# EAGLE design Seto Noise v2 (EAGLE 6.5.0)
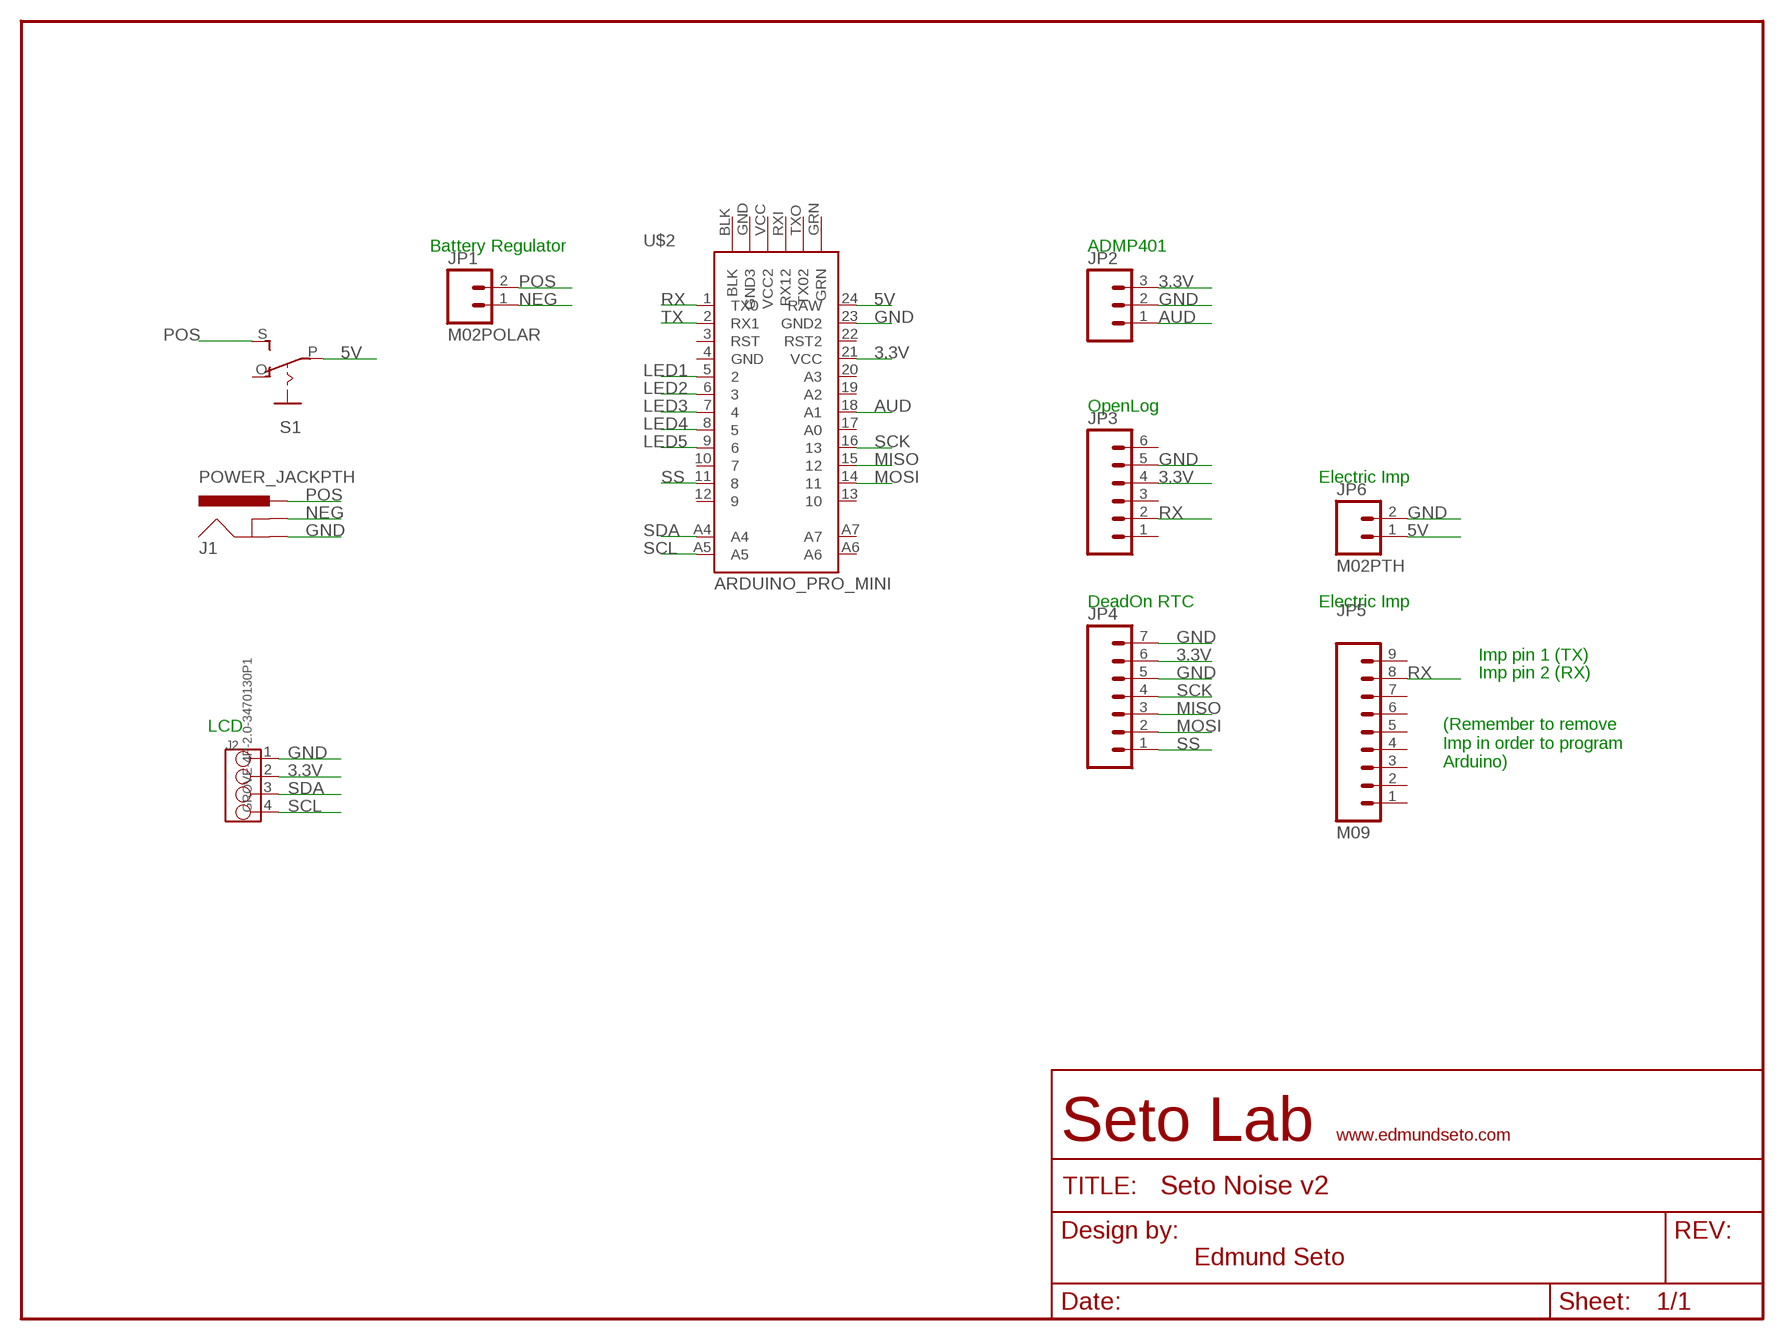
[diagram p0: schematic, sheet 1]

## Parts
J1  POWER_JACKPTH  [POWER_JACK_PTH]
J2  GROVE-4P-2.0-3470130P1  [4P-2.0]
JP1  M02POLAR  [MOLEX-1X2]
JP2  M03PTH  [1X03]
JP3  M06SIP  [1X06]
JP4  M07  [1X07]
JP5  M09  [1X09]
JP6  M02PTH  [1X02]
S1  EG1218S  [EG1218]
U$2  ARDUINO_PRO_MINI  [ARDUINO_PRO_MINI]

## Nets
3.3V: J2.2 JP2.3 JP3.4 JP4.6 U$2.21(VCC)
5V: JP6.1 S1.P U$2.24(RAW)
AUD: JP2.1 U$2.18(A1)
GND: J1.GND J2.1 JP2.2 JP3.5 JP4.5 JP4.7 JP6.2 U$2.23(GND2)
LED1: U$2.5
LED2: U$2.6
LED3: U$2.7
LED4: U$2.8
LED5: U$2.9
MISO: JP4.3 U$2.15
MOSI: JP4.2 U$2.14
NEG: J1.GNDBREAK JP1.1
POS: J1.PWR JP1.2 S1.S
RX: JP3.2 JP5.8 U$2.1(TX0)
SCK: JP4.4 U$2.16
SCL: J2.4 U$2.A5
SDA: J2.3 U$2.A4
SS: JP4.1 U$2.11
TX: U$2.2(RX1)
Unconnected: JP3.1 JP3.3 JP3.6 JP5.1 JP5.2 JP5.3 JP5.4 JP5.5 JP5.6 JP5.7 JP5.9 S1.O U$2.3(RST) U$2.4(GND) U$2.10 U$2.12 U$2.13 U$2.17(A0) U$2.19(A2) U$2.20(A3) U$2.22(RST2) U$2.A6 U$2.A7 U$2.BLK U$2.GND(GND3) U$2.GRN U$2.RXI(RX12) U$2.TXO(TX02) U$2.VCC(VCC2)

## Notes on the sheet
- Battery Regulator | ADMP401
- OpenLog
- Electric Imp
- DeadOn RTC | Electric Imp
- Imp pin 1 (TX)
- Imp pin 2 (RX)
- LCD
- (Remember to remove 
  Imp in order to program 
  Arduino)

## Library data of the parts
J1 = SparkFun-Connectors:POWER_JACK: Power Jack This is the standard 5.5mm barrel jack for power. The PTH is the most common, proven, reliable, footprint. The Slot footprint only works if the mill layer is transmitted to the PCB fab house so be warned. Spark Fun Electronics SKU : PRT-00119 SMT: CONN-08106 Mating wall wart : TOL-00298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
J2 = OPL Eagle Library:GROVE-4P-2.0
JP1 JP6 = SparkFun-Connectors:M02: Standard 2-pin 0.1" header. Use with
JP2 = SparkFun-Connectors:M03: Header 3 Standard 3-pin 0.1" header. Use with straight break away headers (SKU : PRT-00116), right angle break away headers (PRT-00553), swiss pins (PRT-00743), machine pins (PRT-00117), and female headers (PRT-00115). Molex polarized connector foot print use with SKU : PRT-08232 with associated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
JP3 = SparkFun-Connectors:M06: Header 6 Standard 6-pin 0.1" header. Use with straight break away headers (SKU : PRT-00116), right angle break away headers (PRT-00553), swiss pins (PRT-00743), machine pins (PRT-00117), and female headers (PRT-00115). Molex polarized connector foot print use with SKU : PRT-08094 with associated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
JP4 = SparkFun-Connectors:M07: Header 7 Standard 7-pin 0.1" header. Use with straight break away headers (SKU : PRT-00116), right angle break away headers (PRT-00553), swiss pins (PRT-00743), machine pins (PRT-00117), and female headers (PRT-00115). NOTES ON THE VARIANTS LOCK and LOCK_LONGPADS... This footprint was designed to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
JP5 = SparkFun-Connectors:M09: Header 9 Standard 9-pin 0.1" header. Use with straight break away headers (SKU : PRT-00116), right angle break away headers (PRT-00553), swiss pins (PRT-00743), machine pins (PRT-00117), and female headers (PRT-00115).
S1 = adafruit:EG1218: SLIDING SWITCH 0.1" spacing through hole, vertical SPDT slide switch http://www.ladyada.net/library/pcb/eaglelibrary.html
U$2 = SparkFun-Boards_ES:ARDUINO_PRO_MINI

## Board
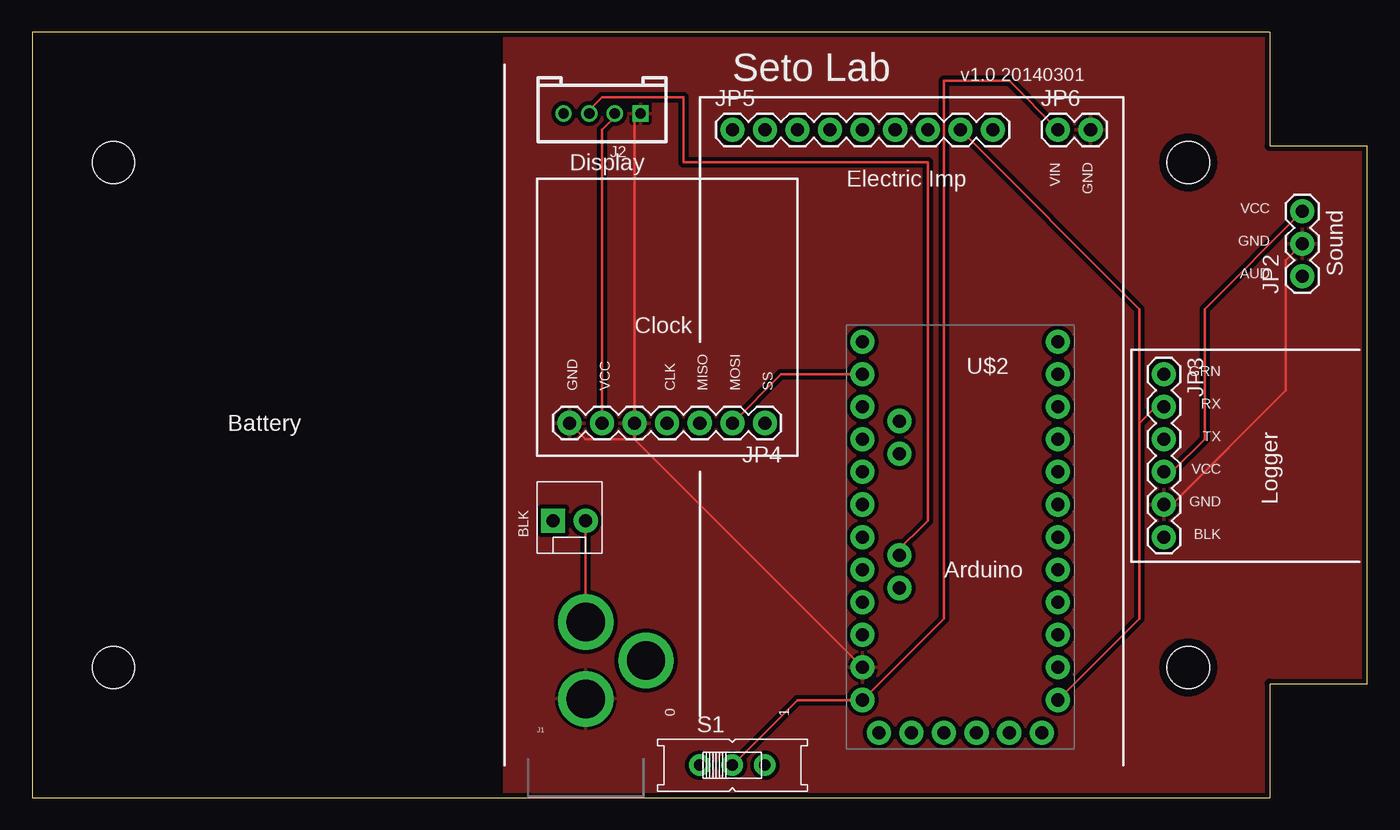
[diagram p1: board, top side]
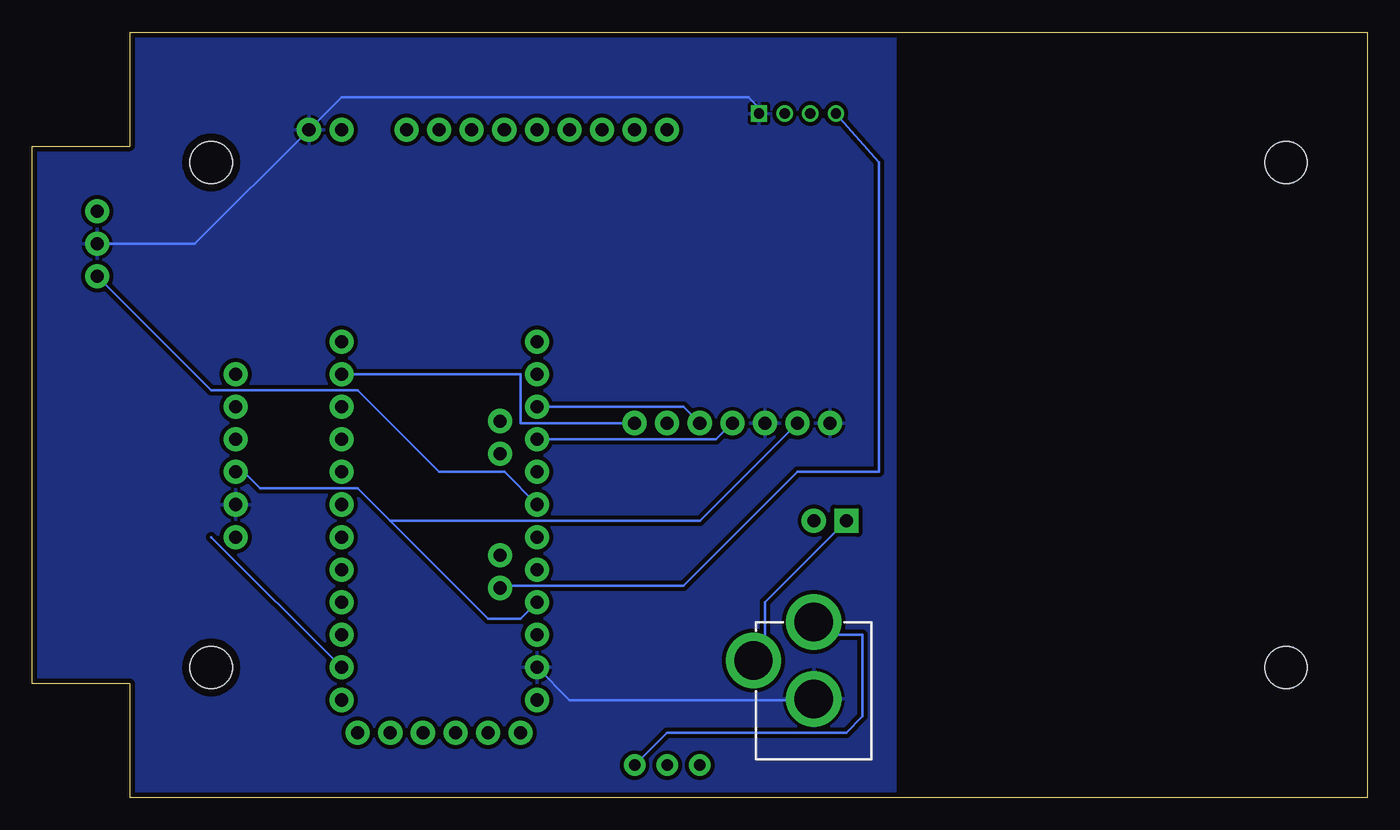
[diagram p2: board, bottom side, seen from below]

Size 104.14 x 59.69 mm. Coordinates in mm from the lower left corner, seen from the top.
Outline: 0,0 96.52,0 96.52,8.89 104.14,8.89 104.14,50.8 96.52,50.8 96.52,59.69 0,59.69 0,0
Copper layers (1*16): Top 0.0356mm / dielectric 1.5011mm / Bottom 0.0356mm
Design rules "LaenPCBOrder": minimum track width 6mil, minimum drill 13mil, track to track 6mil, track to pad 6mil, pad to pad 6mil, via to via 6mil, smd to smd 6mil, copper to edge 15mil, drill to drill 6mil, minimum pad ring 7mil, minimum via ring 7mil, stop-mask expansion 3mil, vias tented up to drill 0mil, thermal gap 10mil

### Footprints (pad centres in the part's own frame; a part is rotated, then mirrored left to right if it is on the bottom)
POWER_JACK_PTH = drill 2.997 pad 4.318: GND 0,7.7; GNDBREAK 4.7,10.7; PWR 0,13.7
4P-2.0 = drill 0.8 pad 1.27 square: 1 -3,0 | drill 0.8 pad 1.27: 2 -1,0; 3 1,0; 4 3,0
MOLEX-1X2 = drill 1.016 pad 1.88 square: 1 0,0 | drill 1.016 pad 1.88: 2 2.54,0
1X03 = drill 1.016 pad 1.88: 1 0,0; 2 2.54,0; 3 5.08,0
1X06 = drill 1.016 pad 1.88: 1 0,0; 2 2.54,0; 3 5.08,0; 4 7.62,0; 5 10.16,0; 6 12.7,0
1X07 = drill 1.016 pad 1.88: 1 0,0; 2 2.54,0; 3 5.08,0; 4 7.62,0; 5 10.16,0; 6 12.7,0; 7 15.24,0
1X09 = drill 1.016 pad 1.88: 1 0,0; 2 2.54,0; 3 5.08,0; 4 7.62,0; 5 10.16,0; 6 12.7,0; 7 15.24,0; 8 17.78,0; 9 20.32,0
1X02 = drill 1.016 pad 1.88: 1 0,0; 2 2.54,0
EG1218 = drill 0.9 pad 1.676: O -2.54,0; P 0,0; S 2.54,0
STAND-OFF = hole 3.302: 0,0
ARDUINO_PRO_MINI = drill 1.016 pad 1.88: 1 -7.62,12.7; 2 -7.62,10.16; 3 -7.62,7.62; 4 -7.62,5.08; 5 -7.62,2.54; 6 -7.62,0; 7 -7.62,-2.54; 8 -7.62,-5.08; 9 -7.62,-7.62; 10 -7.62,-10.16; 11 -7.62,-12.7; 12 -7.62,-15.24; 13 7.62,-15.24; 14 7.62,-12.7; 15 7.62,-10.16; 16 7.62,-7.62; 17 7.62,-5.08; 18 7.62,-2.54; 19 7.62,0; 20 7.62,2.54; 21 7.62,5.08; 22 7.62,7.62; 23 7.62,10.16; 24 7.62,12.7; A4 4.763,1.429; A5 4.763,3.969; A6 4.763,-9.049; A7 4.763,-6.509; BLK -6.35,15.24; GND -3.81,15.24; GRN 6.35,15.24; RXI 1.27,15.24; TXO 3.81,15.24; VCC -1.27,15.24

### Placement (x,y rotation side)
J1  43.18,0 0 top
J2  44.45,53.34 180 top
JP1  40.64,21.59 0 top
JP2  99.06,40.64 90 top
JP3  88.27,33.02 270 top
JP4  57.15,29.21 180 top
JP5  54.61,52.07 0 top
JP6  80.01,52.07 0 top
S1  54.61,2.54 0 top
U$1  [STAND-OFF]  90.17,10.16 0 top
U$2  72.39,20.32 180 top
U$3  [STAND-OFF]  6.35,49.53 0 top
U$4  [STAND-OFF]  6.35,10.16 0 top
U$5  [STAND-OFF]  90.17,49.53 0 top

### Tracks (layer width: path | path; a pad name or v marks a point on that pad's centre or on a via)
3.3V
  Top 0.203: JP4.6 44.45,52.07 45.72,53.34 J2.2 | JP2.3 91.44,38.1 91.44,27.94 88.9,25.4 JP3.4
  Bottom 0.203: U$2.21 66.04,13.97 68.58,13.97 76.2,21.59 | 76.2,21.59 78.74,24.13 86.36,24.13 87.63,25.4 JP3.4 | JP4.6 52.07,21.59 76.2,21.59
5V
  Top 0.203: S1.P 59.69,7.62 U$2.24 71.12,13.97 71.12,55.88 76.2,55.88 JP6.1
AUD
  Bottom 0.203: U$2.18 67.31,25.4 72.39,25.4 78.74,31.75 90.17,31.75 JP2.1
GND
  Top 0.203: JP2.2 97.79,41.91 97.79,31.75 88.9,22.86 JP3.5 | J2.1 46.99,53.34 JP4.5 46.99,27.94 | JP4.7 43.18,27.94 46.99,27.94 | U$2.23 46.99,27.94
  Bottom 0.203: JP2.2 91.44,43.18 JP6.2 80.01,54.61 48.26,54.61 47.45,53.8 J2.1 46.99,53.34 | U$2.23 62.23,7.62 43.18,7.62 J1.GND
  pour Bottom (isolate 0.305): 36.83,0 36.83,59.69 96.52,59.69 96.52,50.8 104.14,50.8 104.14,8.89 96.52,8.89 96.52,0
  pour Top (isolate 0.305): 36.83,0 36.83,59.69 96.52,59.69 96.52,50.8 104.14,50.8 104.14,8.89 96.52,8.89 96.52,0
MISO
  Bottom 0.203: JP4.3 53.34,30.48 U$2.15
MOSI
  Top 0.203: JP4.2 58.42,33.02 U$2.14
NEG
  Bottom 0.203: JP1.1 46.99,15.24 46.99,11.43 J1.GNDBREAK
POS
  Top 0.203: J1.PWR JP1.2
  Bottom 0.203: S1.S 54.61,5.08 40.64,5.08 39.37,6.35 39.37,12.7 43.18,12.7 J1.PWR
RX
  Top 0.203: U$2.1 86.36,13.97 86.36,29.21 | 86.36,29.21 87.63,30.48 JP3.2 | JP5.8 86.36,38.1 86.36,29.21
SCK
  Bottom 0.203: JP4.4 50.8,27.94 U$2.16
SCL
  Bottom 0.203: J2.4 38.1,49.53 38.1,25.4 44.45,25.4 53.34,16.51 67.31,16.51 U$2.A5
SDA
  Top 0.203: J2.3 43.18,53.34 44.45,54.61 50.8,54.61 50.8,49.53 69.85,49.53 69.85,21.59 67.31,19.05 U$2.A4
SS
  Bottom 0.203: JP4.1 66.04,29.21 66.04,33.02 U$2.11
TX
  Bottom 0.203: 90.17,20.32 U$2.2

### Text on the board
tPlace: Seto Lab | v1.0 20140301 | VIN | GND | Display | Electric Imp | VCC | GND | AUD | Sound | Clock | GRN | GND | VCC | CLK | MISO | MOSI | SS | RX | Battery | TX | VCC | GND | Logger | BLK | BLK | Arduino | 0 | 1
